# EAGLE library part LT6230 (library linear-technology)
215MHz, Rail-to-Rail Output, 1.1nV/Hz, 3.5mA Op Amp Source: http://cds.linear.com/docs/Datasheet/623012fb.pdf
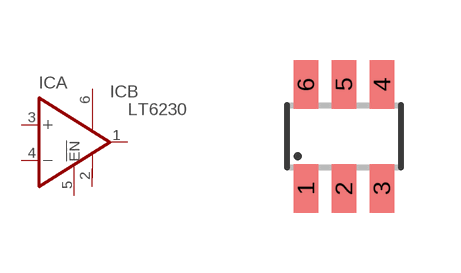
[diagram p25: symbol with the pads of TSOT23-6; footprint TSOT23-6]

Designator prefix IC; gates A=OPAMP-EN B=V+-

## LT6230CS6 (MPN: LT6230CS6#TR; OC_FARNELL: 1663845; OC_NEWARK: 57M9332), LT6230CS6-10 (MPN: LT6230CS6-10#TR; OC_FARNELL: 1663846; OC_NEWARK: 57M9328), LT6230IS6 (MPN: LT6230IS6#TR; OC_FARNELL: unknown; OC_NEWARK: 57M9340), LT6230IS6-10 (MPN: LT6230IS6-10#TR; OC_FARNELL: unknown; OC_NEWARK: 57M9336)  [TSOT23-6]
1  A:OUT  out
2  B:V-  pwr
3  A:+IN  in
4  A:-IN  in
5  A:!EN
6  B:V+  pwr

## Footprint TSOT23-6 (pad centres in mm)
S6 Package 6-Lead Plastic TSOT-23 Source: http://cds.linear.com/docs/Datasheet/623012fb.pdf
smd 0.62 x 1.22: 1 -0.95,-1.3; 2 0,-1.3; 3 0.95,-1.3; 4 0.95,1.3; 5 0,1.3; 6 -0.95,1.3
